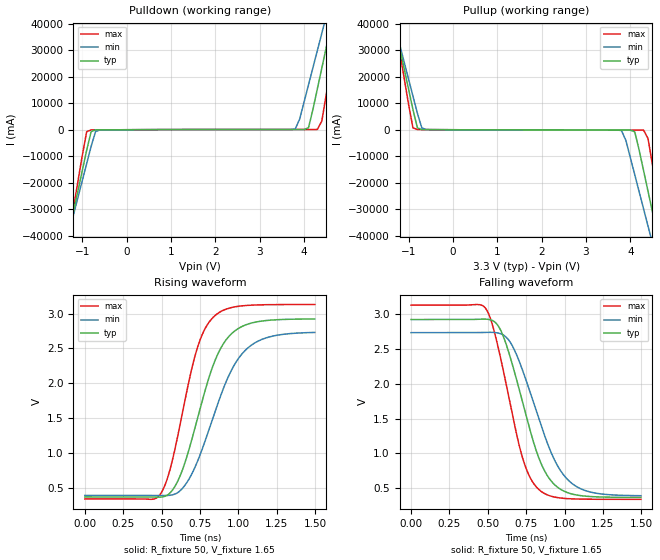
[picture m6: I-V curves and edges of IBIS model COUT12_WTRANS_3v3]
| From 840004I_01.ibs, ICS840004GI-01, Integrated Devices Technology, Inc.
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[Model] COUT12_WTRANS_3v3
Model_type   Output
Polarity   Non-Inverting
|   typ   min   max
C_comp   2pF   1.5pF   2.5pF
Vmeas = 1.65V
Rref = 50
Cref = 0
Vref = 1.65V
|   typ   min   max
[Voltage range]   3.3V   3.135V   3.465V
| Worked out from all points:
|   slope of the pulldown table from 0 to 0.495 V, typ, clamps not added: 14.9 ohm
|   slope of the pullup table from 0 to 0.495 V, typ, clamps not added: 15.2 ohm
|   rising waveform, R_fixture 50, V_fixture 1.65: 20-80 % time 210ps typ, 244ps min, 172ps max; typ from 0.368 V to 2.92 V
|   falling waveform, R_fixture 50, V_fixture 1.65: 20-80 % time 201ps typ, 231ps min, 169ps max; typ from 2.92 V to 0.368 V
[Pulldown]
|Voltage   I (typ)   I (min)   I (max)
-3.3V     -194.8A    -168.6A    -239A
-1.3V     -38.86A    -38.7A     -39.66A
-900mV    -7.663A    -12.73A    -714mA
-800mV    -729.6mA   -6.238A    -72.99mA
-600mV    -42.99mA   -63.63mA   -47.95mA
3.8V      78.05mA    271.7mA    90.74mA
4.1V      746.8mA    16.95A     91.13mA
4.3V      15.46A     29.92A     116.8mA
4.4V      23.25A     36.41A     3.273A
4.6V      38.83A     49.38A     23.19A
4.8V      54.42A     62.36A     43.12A
6.6V      194.8A     179.2A     222.5A
[Pullup]
|Voltage   I (typ)   I (min)   I (max)
-3.3V     194.8A     168.6A     239.1A
-1.3V     38.84A     38.69A     39.64A
-900mV    7.659A     12.72A     713.3mA
-800mV    728.1mA    6.236A     76.49mA
-600mV    45.44mA    64.77mA    54.17mA
3.8V      -101.2mA   -294.2mA   -125.1mA
4.1V      -781.9mA   -16.99A    -128.9mA
4.3V      -15.51A    -29.97A    -167.7mA
4.4V      -23.31A    -36.46A    -3.333A
4.6V      -38.9A     -49.45A    -23.27A
4.8V      -54.5A     -62.43A    -43.21A
6.6V      -194.9A    -179.3A    -222.7A
[Ramp]
|   typ   min   max
dV/dt_r   2.047/0.326n   1.873/0.378n   2.238/0.266n
dV/dt_f   2.05/0.303n   1.879/0.349n   2.24/0.255n
R_load =   50.0000
[Rising Waveform]
R_fixture = 50
V_fixture = 1.65   |Vcc_typ
V_fixture_min = 1.5675 |Vcc_min
V_fixture_max = 1.7325 |Vcc_max
C_fixture = 0.0p
| Time   typ   min   max
0s        367.7mV    389.5mV    340.1mV
491ps     365.1mV    388.9mV    404.4mV
552.6ps   419.2mV    391mV      741.5mV
626.1ps   699.7mV    467.9mV    1.469V
738.7ps   1.533V     903.8mV    2.545V
851.4ps   2.343V     1.609V     2.978V
961ps     2.722V     2.211V     3.09V
1.074ns   2.857V     2.528V     3.12V
1.228ns   2.909V     2.679V     3.129V
1.498ns   2.923V     2.73V      3.131V
[Falling Waveform]
R_fixture = 50
V_fixture = 1.65   |Vcc_typ
V_fixture_min = 1.5675 |Vcc_min
V_fixture_max = 1.7325 |Vcc_max
C_fixture = 0.0p
| Time   typ   min   max
0s        2.925V     2.736V     3.131V
488ps     2.93V      2.74V      3.078V
572.1ps   2.818V     2.728V     2.48V
650.1ps   2.353V     2.584V     1.668V
740.2ps   1.624V     2.11V      840.5mV
837.8ps   905.1mV    1.466V     471.1mV
944.4ps   532.5mV    863.6mV    368.6mV
1.056ns   412.8mV    556.5mV    346.2mV
1.206ns   376mV      428mV      340.9mV
1.498ns   368.1mV    392.2mV    340.1mV
